DATA_BLOCK DB 99
TITLE = Main data block
VERSION : 0.1
STRUCT
	VAR0	: ARRAY  [1 .. 2] OF INT;
	VAR1	: ARRAY  [1 .. 2] OF INT  := 1, 2;
	VAR2	: ARRAY  [1 .. 2, 1 .. 2] OF INT  := 1, 2, 3, 4;
	VAR3	: ARRAY  [-2 .. -1] OF INT := -2, -1;
	VAR4	: ARRAY  [1 .. 2, 1 .. 2, 1 .. 2, 1 .. 2, 1 .. 2, 1 .. 2] OF INT := 4 (1, 2, 3, 4, 5, 6, 7, 8, 9, 10, 11, 12, 13, 14, 15, 16);
	VAR5	: ARRAY  [0 .. 9 ] OF INT := 5 (1, 2);
	VAR6	: ARRAY  [1 .. 2, 1 .. 10, 1 .. 5 ] OF INT := 5 (1, 2, 3, 4, 5, 6, 7, 8, 9, 10, 11, 12, 13, 14, 15, 16, 17, 18, 19, 20);
	VAR7	: ARRAY  [1 .. 14 ] OF BOOL := 7 (TRUE, FALSE);
	VAR8	: ARRAY  [1 .. 3 ] OF BOOL := TRUE, FALSE, TRUE;
	VAR9	: ARRAY  [1 .. 1 ] OF INT := 42;
//	VAR10	: STRUCT
//		VAR10_1		: INT  := 101;
//		VAR10_2		: ARRAY  [1 .. 2 ] OF INT  := 1, 2;
//		VAR10_3		: ARRAY  [1 .. 2 ] OF STRUCT
//			VAR10_3_1	: INT  := 1031;
//			VAR10_3_2	: ARRAY  [1 .. 2 ] OF INT  := 1, 2;
//		END_STRUCT;
//	END_STRUCT;
END_STRUCT;
BEGIN
	VAR0[1]				:= 0;
	VAR0[2]				:= 0;
	VAR1[1]				:= -30000;
	VAR1[2]				:= 30000;
	VAR2[1, 1]			:= 1;
	VAR2[1, 2]			:= 2;
	VAR2[2, 1]			:= 3;
	VAR2[2, 2]			:= 4;
	VAR3[-2]			:= -2;
	VAR3[-1]			:= -1;
	VAR4[1, 1, 1, 1, 1, 1]		:= 1;
	VAR4[1, 1, 1, 1, 1, 2]		:= 2;
	VAR4[1, 1, 1, 1, 2, 1]		:= 3;
	VAR4[1, 1, 1, 1, 2, 2]		:= 4;
	VAR4[1, 1, 1, 2, 1, 1]		:= 5;
	VAR4[1, 1, 1, 2, 1, 2]		:= 6;
	VAR4[1, 1, 1, 2, 2, 1]		:= 7;
	VAR4[1, 1, 1, 2, 2, 2]		:= 8;
	VAR4[1, 1, 2, 1, 1, 1]		:= 9;
	VAR4[1, 1, 2, 1, 1, 2]		:= 10;
	VAR4[1, 1, 2, 1, 2, 1]		:= 11;
	VAR4[1, 1, 2, 1, 2, 2]		:= 12;
	VAR4[1, 1, 2, 2, 1, 1]		:= 13;
	VAR4[1, 1, 2, 2, 1, 2]		:= 14;
	VAR4[1, 1, 2, 2, 2, 1]		:= 15;
	VAR4[1, 1, 2, 2, 2, 2]		:= 16;
	VAR4[1, 2, 1, 1, 1, 1]		:= 1;
	VAR4[1, 2, 1, 1, 1, 2]		:= 2;
	VAR4[1, 2, 1, 1, 2, 1]		:= 3;
	VAR4[1, 2, 1, 1, 2, 2]		:= 4;
	VAR4[1, 2, 1, 2, 1, 1]		:= 5;
	VAR4[1, 2, 1, 2, 1, 2]		:= 6;
	VAR4[1, 2, 1, 2, 2, 1]		:= 7;
	VAR4[1, 2, 1, 2, 2, 2]		:= 8;
	VAR4[1, 2, 2, 1, 1, 1]		:= 9;
	VAR4[1, 2, 2, 1, 1, 2]		:= 10;
	VAR4[1, 2, 2, 1, 2, 1]		:= 11;
	VAR4[1, 2, 2, 1, 2, 2]		:= 12;
	VAR4[1, 2, 2, 2, 1, 1]		:= 13;
	VAR4[1, 2, 2, 2, 1, 2]		:= 14;
	VAR4[1, 2, 2, 2, 2, 1]		:= 15;
	VAR4[1, 2, 2, 2, 2, 2]		:= 16;
	VAR4[2, 1, 1, 1, 1, 1]		:= 1;
	VAR4[2, 1, 1, 1, 1, 2]		:= 2;
	VAR4[2, 1, 1, 1, 2, 1]		:= 3;
	VAR4[2, 1, 1, 1, 2, 2]		:= 4;
	VAR4[2, 1, 1, 2, 1, 1]		:= 5;
	VAR4[2, 1, 1, 2, 1, 2]		:= 6;
	VAR4[2, 1, 1, 2, 2, 1]		:= 7;
	VAR4[2, 1, 1, 2, 2, 2]		:= 8;
	VAR4[2, 1, 2, 1, 1, 1]		:= 9;
	VAR4[2, 1, 2, 1, 1, 2]		:= 10;
	VAR4[2, 1, 2, 1, 2, 1]		:= 11;
	VAR4[2, 1, 2, 1, 2, 2]		:= 12;
	VAR4[2, 1, 2, 2, 1, 1]		:= 13;
	VAR4[2, 1, 2, 2, 1, 2]		:= 14;
	VAR4[2, 1, 2, 2, 2, 1]		:= 15;
	VAR4[2, 1, 2, 2, 2, 2]		:= 16;
	VAR4[2, 2, 1, 1, 1, 1]		:= 1;
	VAR4[2, 2, 1, 1, 1, 2]		:= 2;
	VAR4[2, 2, 1, 1, 2, 1]		:= 3;
	VAR4[2, 2, 1, 1, 2, 2]		:= 4;
	VAR4[2, 2, 1, 2, 1, 1]		:= 5;
	VAR4[2, 2, 1, 2, 1, 2]		:= 6;
	VAR4[2, 2, 1, 2, 2, 1]		:= 7;
	VAR4[2, 2, 1, 2, 2, 2]		:= 8;
	VAR4[2, 2, 2, 1, 1, 1]		:= 9;
	VAR4[2, 2, 2, 1, 1, 2]		:= 10;
	VAR4[2, 2, 2, 1, 2, 1]		:= 11;
	VAR4[2, 2, 2, 1, 2, 2]		:= 12;
	VAR4[2, 2, 2, 2, 1, 1]		:= 13;
	VAR4[2, 2, 2, 2, 1, 2]		:= 14;
	VAR4[2, 2, 2, 2, 2, 1]		:= 15;
	VAR4[2, 2, 2, 2, 2, 2]		:= 16;
	VAR5[0]				:= 1;
	VAR5[1]				:= 2;
	VAR5[2]				:= 1;
	VAR5[3]				:= 2;
	VAR5[4]				:= 1;
	VAR5[5]				:= 2;
	VAR5[6]				:= 1;
	VAR5[7]				:= 2;
	VAR5[8]				:= 1;
	VAR5[9]				:= 2;
	VAR6[1, 1, 1]			:= 1;
	VAR6[1, 1, 2]			:= 2;
	VAR6[1, 1, 3]			:= 3;
	VAR6[1, 1, 4]			:= 4;
	VAR6[1, 1, 5]			:= 5;
	VAR6[1, 2, 1]			:= 6;
	VAR6[1, 2, 2]			:= 7;
	VAR6[1, 2, 3]			:= 8;
	VAR6[1, 2, 4]			:= 9;
	VAR6[1, 2, 5]			:= 10;
	VAR6[1, 3, 1]			:= 11;
	VAR6[1, 3, 2]			:= 12;
	VAR6[1, 3, 3]			:= 13;
	VAR6[1, 3, 4]			:= 14;
	VAR6[1, 3, 5]			:= 15;
	VAR6[1, 4, 1]			:= 16;
	VAR6[1, 4, 2]			:= 17;
	VAR6[1, 4, 3]			:= 18;
	VAR6[1, 4, 4]			:= 19;
	VAR6[1, 4, 5]			:= 20;
	VAR6[1, 5, 1]			:= 1;
	VAR6[1, 5, 2]			:= 2;
	VAR6[1, 5, 3]			:= 3;
	VAR6[1, 5, 4]			:= 4;
	VAR6[1, 5, 5]			:= 5;
	VAR6[1, 6, 1]			:= 6;
	VAR6[1, 6, 2]			:= 7;
	VAR6[1, 6, 3]			:= 8;
	VAR6[1, 6, 4]			:= 9;
	VAR6[1, 6, 5]			:= 10;
	VAR6[1, 7, 1]			:= 11;
	VAR6[1, 7, 2]			:= 12;
	VAR6[1, 7, 3]			:= 13;
	VAR6[1, 7, 4]			:= 14;
	VAR6[1, 7, 5]			:= 15;
	VAR6[1, 8, 1]			:= 16;
	VAR6[1, 8, 2]			:= 17;
	VAR6[1, 8, 3]			:= 18;
	VAR6[1, 8, 4]			:= 19;
	VAR6[1, 8, 5]			:= 20;
	VAR6[1, 9, 1]			:= 1;
	VAR6[1, 9, 2]			:= 2;
	VAR6[1, 9, 3]			:= 3;
	VAR6[1, 9, 4]			:= 4;
	VAR6[1, 9, 5]			:= 5;
	VAR6[1, 10, 1]			:= 6;
	VAR6[1, 10, 2]			:= 7;
	VAR6[1, 10, 3]			:= 8;
	VAR6[1, 10, 4]			:= 9;
	VAR6[1, 10, 5]			:= 10;
	VAR6[2, 1, 1]			:= 11;
	VAR6[2, 1, 2]			:= 12;
	VAR6[2, 1, 3]			:= 13;
	VAR6[2, 1, 4]			:= 14;
	VAR6[2, 1, 5]			:= 15;
	VAR6[2, 2, 1]			:= 16;
	VAR6[2, 2, 2]			:= 17;
	VAR6[2, 2, 3]			:= 18;
	VAR6[2, 2, 4]			:= 19;
	VAR6[2, 2, 5]			:= 20;
	VAR6[2, 3, 1]			:= 1;
	VAR6[2, 3, 2]			:= 2;
	VAR6[2, 3, 3]			:= 3;
	VAR6[2, 3, 4]			:= 4;
	VAR6[2, 3, 5]			:= 5;
	VAR6[2, 4, 1]			:= 6;
	VAR6[2, 4, 2]			:= 7;
	VAR6[2, 4, 3]			:= 8;
	VAR6[2, 4, 4]			:= 9;
	VAR6[2, 4, 5]			:= 10;
	VAR6[2, 5, 1]			:= 11;
	VAR6[2, 5, 2]			:= 12;
	VAR6[2, 5, 3]			:= 13;
	VAR6[2, 5, 4]			:= 14;
	VAR6[2, 5, 5]			:= 15;
	VAR6[2, 6, 1]			:= 16;
	VAR6[2, 6, 2]			:= 17;
	VAR6[2, 6, 3]			:= 18;
	VAR6[2, 6, 4]			:= 19;
	VAR6[2, 6, 5]			:= 20;
	VAR6[2, 7, 1]			:= 1;
	VAR6[2, 7, 2]			:= 2;
	VAR6[2, 7, 3]			:= 3;
	VAR6[2, 7, 4]			:= 4;
	VAR6[2, 7, 5]			:= 5;
	VAR6[2, 8, 1]			:= 6;
	VAR6[2, 8, 2]			:= 7;
	VAR6[2, 8, 3]			:= 8;
	VAR6[2, 8, 4]			:= 9;
	VAR6[2, 8, 5]			:= 10;
	VAR6[2, 9, 1]			:= 11;
	VAR6[2, 9, 2]			:= 12;
	VAR6[2, 9, 3]			:= 13;
	VAR6[2, 9, 4]			:= 14;
	VAR6[2, 9, 5]			:= 15;
	VAR6[2, 10, 1]			:= 16;
	VAR6[2, 10, 2]			:= 17;
	VAR6[2, 10, 3]			:= 18;
	VAR6[2, 10, 4]			:= 19;
	VAR6[2, 10, 5]			:= 20;
	VAR7[1]				:= TRUE;
	VAR7[2]				:= FALSE;
	VAR7[3]				:= TRUE;
	VAR7[4]				:= FALSE;
	VAR7[5]				:= TRUE;
	VAR7[6]				:= FALSE;
	VAR7[7]				:= TRUE;
	VAR7[8]				:= FALSE;
	VAR7[9]				:= TRUE;
	VAR7[10]			:= FALSE;
	VAR7[11]			:= TRUE;
	VAR7[12]			:= FALSE;
	VAR7[13]			:= TRUE;
	VAR7[14]			:= FALSE;
	VAR8[1]				:= TRUE;
	VAR8[2]				:= FALSE;
	VAR8[3]				:= TRUE;
	VAR9[1]				:= 42;
//	VAR10.VAR10_1			:= 101;
//	VAR10.VAR10_2[1]		:= 1;
//	VAR10.VAR10_2[2]		:= 2;
//	VAR10.VAR10_3[1].VAR10_3_1	:= 1031;
//	VAR10.VAR10_3[1].VAR10_3_2[1]	:= 1;
//	VAR10.VAR10_3[1].VAR10_3_2[2]	:= 2;
//	VAR10.VAR10_3[2].VAR10_3_1	:= 1031;
//	VAR10.VAR10_3[2].VAR10_3_2[1]	:= 1;
//	VAR10.VAR10_3[2].VAR10_3_2[2]	:= 2;
END_DATA_BLOCK


FUNCTION_BLOCK FB 1
VAR_INPUT
	VAR0	: ARRAY [1 .. 2] OF INT;
	VAR1	: ARRAY [1 .. 2, 0 .. 1] OF INT;
	SELECT	: INT;
END_VAR
BEGIN
	L		#SELECT
	SPL		ERR
	SPA		M000
	SPA		M001
ERR:	__ASSERT==	1,		2	// Wrong #SELECT


	// Check instance-DB initial values
M000:	L		#VAR0[1]
	__ASSERT==	__ACCU 1,	1
	L		DIW 0
	__ASSERT==	__ACCU 1,	1
	L		#VAR0[2]
	__ASSERT==	__ACCU 1,	2
	L		DIW 2
	__ASSERT==	__ACCU 1,	2
	L		#VAR1[1, 0]
	__ASSERT==	__ACCU 1,	100
	L		DIW 4
	__ASSERT==	__ACCU 1,	100
	L		#VAR1[1, 1]
	__ASSERT==	__ACCU 1,	101
	L		DIW 6
	__ASSERT==	__ACCU 1,	101
	L		#VAR1[2, 0]
	__ASSERT==	__ACCU 1,	102
	L		DIW 8
	__ASSERT==	__ACCU 1,	102
	L		#VAR1[2, 1]
	__ASSERT==	__ACCU 1,	103
	L		DIW 10
	__ASSERT==	__ACCU 1,	103

	L		P##VAR0 // Ptr to array name is ptr to first element
	__ASSERT==	__ACCU 1,	DW#16#85000000
	LAR1
	L		W [AR1, P#0.0]
	__ASSERT==	__ACCU 1,	1

	BEA


	// Check passed parameters
M001:	L		#VAR0[1]
	__ASSERT==	__ACCU 1,	91
	L		DIW 0
	__ASSERT==	__ACCU 1,	91
	L		#VAR0[2]
	__ASSERT==	__ACCU 1,	92
	L		DIW 2
	__ASSERT==	__ACCU 1,	92
	L		#VAR1[1, 0]
	__ASSERT==	__ACCU 1,	9100
	L		DIW 4
	__ASSERT==	__ACCU 1,	9100
	L		#VAR1[1, 1]
	__ASSERT==	__ACCU 1,	9101
	L		DIW 6
	__ASSERT==	__ACCU 1,	9101
	L		#VAR1[2, 0]
	__ASSERT==	__ACCU 1,	9102
	L		DIW 8
	__ASSERT==	__ACCU 1,	9102
	L		#VAR1[2, 1]
	__ASSERT==	__ACCU 1,	9103
	L		DIW 10
	__ASSERT==	__ACCU 1,	9103

	L		P##VAR0 // Ptr to array name is ptr to first element
	__ASSERT==	__ACCU 1,	DW#16#85000000
	LAR1
	L		W [AR1, P#0.0]
	__ASSERT==	__ACCU 1,	91

	BEA

END_FUNCTION_BLOCK


DATA_BLOCK DB 1
TITLE = FB 1 instance DB
FB 1
BEGIN
	VAR0[1]		:= 1;
	VAR0[2]		:= 2;
	VAR1[1, 0]	:= 100;
	VAR1[1, 1]	:= 101;
	VAR1[2, 0]	:= 102;
	VAR1[2, 1]	:= 103;
	SELECT		:= 0;
END_DATA_BLOCK

DATA_BLOCK DB 2
TITLE = FB 1 parameter passing DB
STRUCT
	VAR0	: ARRAY [1 .. 2] OF INT;
	VAR1	: ARRAY [1 .. 2, 0 .. 1] OF INT;
END_STRUCT
BEGIN
	VAR0[1]		:= 91;
	VAR0[2]		:= 92;
	VAR1[1, 0]	:= 9100;
	VAR1[1, 1]	:= 9101;
	VAR1[2, 0]	:= 9102;
	VAR1[2, 1]	:= 9103;
END_DATA_BLOCK


ORGANIZATION_BLOCK OB 1
BEGIN

	// Check DB99 initial values
	L		DB99.VAR0[1]
	__ASSERT==	__ACCU 1,	0
	L		DB99.DBW 0
	__ASSERT==	__ACCU 1,	0
	L		DB99.VAR0[2]
	__ASSERT==	__ACCU 1,	0
	L		DB99.DBW 2
	__ASSERT==	__ACCU 1,	0
	L		DB99.VAR1[1]
	__ASSERT==	__ACCU 1,	-30000
	L		DB99.DBW 4
	__ASSERT==	__ACCU 1,	-30000
	L		DB99.VAR1[2]
	__ASSERT==	__ACCU 1,	30000
	L		DB99.DBW 6
	__ASSERT==	__ACCU 1,	30000
	L		DB99.VAR2[1, 1]
	__ASSERT==	__ACCU 1,	1
	L		DB99.DBW 8
	__ASSERT==	__ACCU 1,	1
	L		DB99.VAR2[1, 2]
	__ASSERT==	__ACCU 1,	2
	L		DB99.DBW 10
	__ASSERT==	__ACCU 1,	2
	L		DB99.VAR2[2, 1]
	__ASSERT==	__ACCU 1,	3
	L		DB99.DBW 12
	__ASSERT==	__ACCU 1,	3
	L		DB99.VAR2[2, 2]
	__ASSERT==	__ACCU 1,	4
	L		DB99.DBW 14
	__ASSERT==	__ACCU 1,	4


	// Call FB 1 without array parameter passing
	CALL FB 1, DB 1 (
		SELECT	:= 0,
	)

	// Call FB 1 with array parameter passing
//TODO	CALL FB 1, DB 1 (
//		VAR0	:= DB2.VAR0,
//		VAR1	:= DB2.VAR1,
//		SELECT	:= 1,
//	)

	//TODO FC-tests


	CALL SFC 46 // STOP CPU
END_ORGANIZATION_BLOCK
